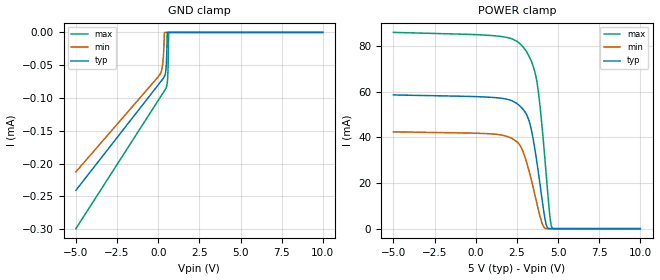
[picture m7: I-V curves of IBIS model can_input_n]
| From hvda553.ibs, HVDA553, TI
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[Model]   can_input_n
Model_type   Input
Vinl = 0.4
Vinh = 1.15
|   typ   min   max
|   (nom PVT)   (fast PVT)   (slow PVT)
 C_comp   7.408e-12   7.174e-12   7.489e-12
| Where nom  PVT is Nominal Process, 5V, 27C
|   Fast PVT is Strong Process,  5.33V, -40C
|   Slow PVT is Weak Process,   4.68V, 150C
[Voltage Range]   5   4.68   5.33
|Junction Temperature
[Temperature Range]   27   150   -40
[Power Clamp Reference]   5   4.68   5.33
[GND Clamp Reference]   0   0   0
[GND Clamp]
|   Voltage   I(typ)   I(min)   I(max)
-5V       -240.6uA   -212.4uA   -299uA
100mV     -76.79uA   -64.23uA   -99.79uA
283.7mV   -70.81uA   -45.78uA   -92.61uA
382mV     -66.81uA   0A         -88.75uA
480mV     -53.57uA   0A         -84.42uA
515mV     -36.55uA   0A         -81.94uA
555mV     0A         0A         -75.96uA
580.5mV   0A         0A         -67.04uA
612.5mV   0A         0A         -40.14uA
633.8mV   0A         0A         -1.309uA
644.5mV   0A         0A         0A
9.995V    0A         0A         0A
[POWER Clamp]
|   Voltage   I(typ)   I(min)   I(max)
-5V       58.59mA    42.42mA    86mA
1.299V    57.36mA    41.32mA    84.42mA
2.565V    54.49mA    37.66mA    81.78mA
2.83V     52.68mA    34.56mA    80.01mA
3.24V     47.37mA    25.27mA    75.55mA
3.453V    40.68mA    19.14mA    71.96mA
3.695V    30.09mA    11.68mA    65.28mA
3.905V    19.47mA    5.441mA    53.76mA
4.225V    3.605mA    150.3uA    28.65mA
4.468V    0A         0A         8.123mA
4.631V    0A         0A         415.5uA
9.995V    0A         0A         0A
